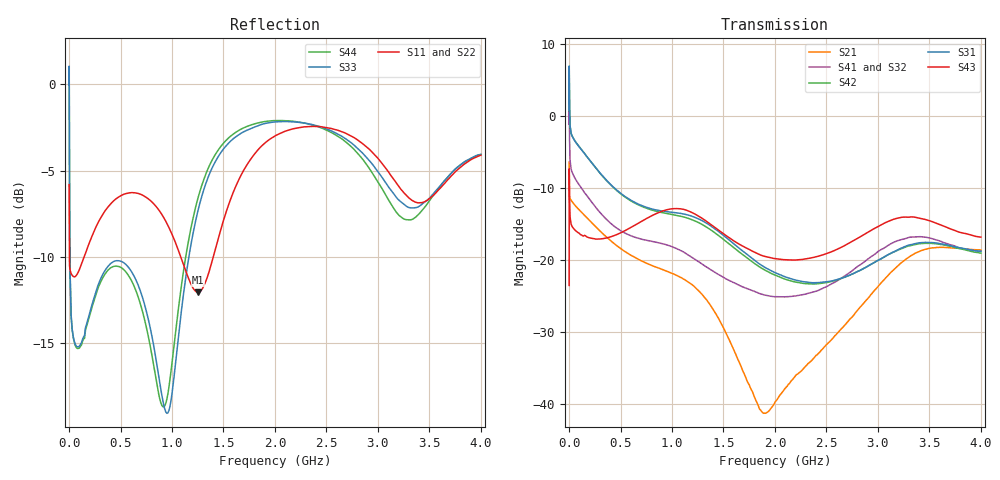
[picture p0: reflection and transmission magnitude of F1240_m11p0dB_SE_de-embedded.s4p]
! Integrated Device Technology
! Corporate Headquarters
! 6024 Silver Creek Valley Road
! San Jose, CA 95138  USA
! Phone:  1-408-284-8200
! Toll Free:  1-800-223-1366
! Webpage:  http://www.idt.com/
! Timing and RF Division
! 515 Groton Road, Suite 102
! Westford, MA 01886-6024
! Device:  F1240
! Description: Dual Intermediate Frequency Digital Variable Gain Amplifier
! Frequency:  10.0 -  500.00 MHz
! Package:  5x5 mm QFN Plastic Package: 32 pin
! Ports:  8 RF, 20 DC
!  Pin  1  = GA3 / Data  Pin 17  = RF OUT_B+
!  Pin  2  = GA4 / CLK  Pin 18  = RF OUT_B-
!  Pin  3  = GA5  Pin 19  = STBY_B
!  Pin  4  = VMODE  Pin 20  = Ground
!  Pin  5  = No Connect  Pin 21  = Ground
!  Pin  6  = GB5  Pin 22  = STB_A
!  Pin  7  = GB4  Pin 23  = RF OUT_A-  = Port 4
!  Pin  8  = GB3  Pin 24  = RF OUT_A+  = Port 3
!  Pin  9  = GB2  Pin 25  = GA0
!  Pin 10  = GB1  Pin 26  = ISET_A
!  Pin 11  = RF IN_B+  Pin 27  = VCC
!  Pin 12  = RF IN_B-  Pin 28  = Ground
!  Pin 13  = Ground  Pin 29  = RF IN_A-  = Port 2
!  Pin 14  = VCC  Pin 30  = RF IN_A+  = Port 1
!  Pin 15  = ISET_B  Pin 31  = GA1
!  Pin 16  = GB0  Pin 32  = GA2 / CSb
! Gain  = +19.5 dB
! State  = 1
! Voltage  = +5.00 V
! Current  = 85.292 mA (one channel only)
! Temperture  =  +25 C
! Test Date  =  2017-10-18
! Board  =  EB4031
! Data:  The device was measured on a custom evaluation board which has
!  individual transmission lines to the RF pins.  Data was collected
!  using a calibrated network analyzer.  The evaluation board was
!  de-embedded using Automatic Fixture Removal.
!  The reference plane is the edge of the package pin.
!  Only Channel A was measured.
!  This data is in single-ended operation.  If your needs are balanced
!  or differential S-parameters then this file needs to be used a
!  linear simulator.
! File Date:  2017-11-10  MJV
! Note:
!  Integrated Device Technology supplies this data as a sample of measured
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# Hz S dB R 100
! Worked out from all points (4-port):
!   410 points, 500 kHz to 4 GHz, reference 100 ohm
!   strongest paths, dB at 500 kHz, 930 MHz, 1.96 GHz, 2.98 GHz, 4 GHz:
!     S43: -23.6, -13.1, -19.7, -15.5, -16.9
!     S31: 0.7, -13.3, -21.5, -20.2, -18.8
!     S42: 0.7, -13.5, -21.9, -20.3, -19.1
!     S41: -1.2, -17.9, -25.1, -19.1, -18.8
!     S32: -1.2, -18.0, -24.9, -19.3, -19.0
!     S21: -6.4, -21.5, -40.6, -24.1, -18.6
!   lowest |S11| = -12.1 dB at 1.25 GHz (marker M1), VSWR 1.66, Z = 60.9 - j9.04 ohm
!   |S11| at or under -10 dB: 3.089 MHz to 148.1 MHz (145.1 MHz wide, 192 % of centre); 1.084 GHz to 1.401 GHz (317.3 MHz wide, 25.5 % of centre)
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500000  -5.82 -5.6  -6.42 -5.8  -31.95 76.4  -33.91 75.7
        -6.43 -5.8  -5.82 -5.6  -33.92 74.7  -31.94 77.5
        0.72 -112.2  -1.16 -113.8  -0.05 -0.4  -23.56 -37.8
        -1.17 -112.7  0.72 -111.1  -23.56 -37.8  -0.06 1.9
3500000  -10.21 -17.1  -11.03 -15.9  -25.75 2.7  -29.78 -11.5
         -11.03 -15.9  -10.21 -17.2  -29.74 -11.8  -25.75 2.9
         2.67 154.1  -1.05 141.0  -4.25 -83.1  -9.60 176.5
         -1.08 141.3  2.67 154.3  -9.60 176.5  -4.29 -83.1
3.6e8  -7.25 -122.5  -16.80 -96.8  -30.67 -78.4  -37.27 -77.1
       -16.79 -96.7  -7.18 -123.3  -37.34 -75.4  -30.85 -78.4
       -8.89 60.6  -14.41 28.9  -10.70 -161.0  -17.02 52.7
       -14.33 28.2  -8.95 59.2  -16.98 52.5  -10.91 -161.8
1.25e9  -12.07 -163.8  -24.27 96.1  -30.17 121.8  -35.45 152.4
        -24.18 96.2  -11.92 -163.4  -35.22 155.7  -31.51 125.3
        -14.27 -134.6  -20.11 153.2  -7.38 -116.6  -14.01 172.5
        -20.20 146.0  -14.79 -135.8  -13.87 172.7  -6.64 -119.3
1.9e9  -3.42 -166.3  -41.01 47.3  -33.52 5.8  -36.15 27.4
       -41.30 45.6  -3.32 -166.9  -36.51 32.9  -34.91 12.6
       -21.03 91.3  -24.66 26.9  -2.27 -173.7  -19.71 53.8
       -24.89 20.2  -21.40 93.9  -19.52 54.8  -2.16 -176.7
2.84e9  -3.39 111.9  -26.39 -7.6  -29.82 -133.4  -32.18 -120.1
        -26.39 -7.5  -3.21 112.4  -32.68 -107.9  -31.09 -124.5
        -21.37 -49.4  -20.78 -125.5  -3.92 105.0  -17.37 -80.2
        -20.58 -136.3  -21.38 -46.0  -16.70 -77.8  -4.26 98.2
4e9  -4.11 -127.6  -18.64 124.7  -27.24 -18.3  -28.33 -3.7
     -18.63 124.8  -3.88 -126.2  -28.92 9.6  -28.94 -7.6
     -18.82 61.2  -19.03 -33.1  -4.06 -132.9  -18.30 61.2
     -18.78 -46.9  -19.08 67.4  -16.85 55.4  -4.07 -142.9
